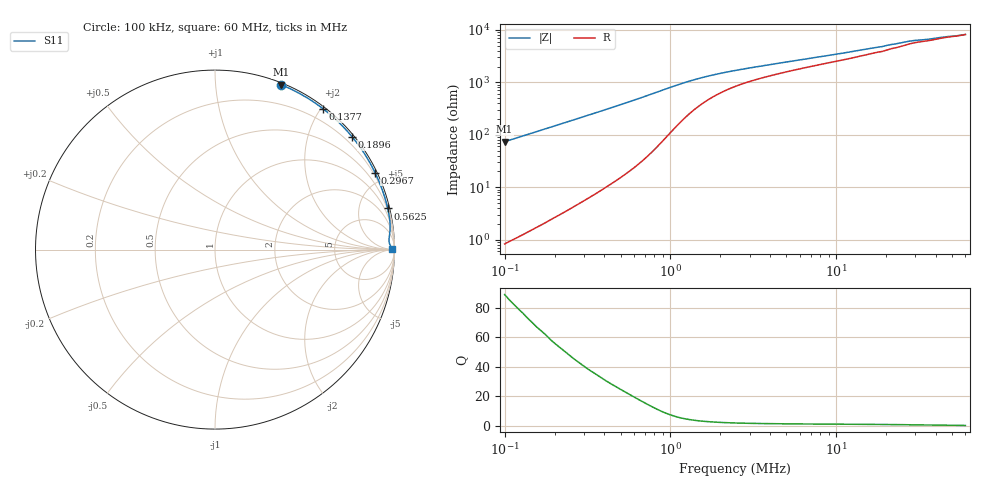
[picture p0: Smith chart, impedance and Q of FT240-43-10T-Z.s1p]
! ListType=Log
!!FT240-43 10T Z
# MHz S RI R 50
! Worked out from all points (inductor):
!   101 points, 100 kHz to 60 MHz, reference 50 ohm
!   read as one part to ground: L = 117 uH near 100 kHz
!   highest Q = 89 at 100 kHz (marker M1), where L = 117 uH
!   S11 on the Smith chart (normalised r, x): 100 kHz: 0.02, +1.47; 137.7 kHz: 0.03, +2.03; 189.6 kHz: 0.05, +2.79; 296.7 kHz: 0.11, +4.38; 562.5 kHz: 0.40, +8.48; 60 MHz: open
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0.1  0.3658 0.9195
0.1136483  0.4694 0.8709
0.1211559  0.5168 0.8436
0.1376916  0.6024 0.7846
0.1564842  0.6759 0.7222
0.1668215  0.7082 0.6906
0.1895899  0.7646 0.6276
0.2021141  0.7889 0.5968
0.2296993  0.8308 0.5372
0.2610494  0.8646 0.481
0.2966783  0.8917 0.4288
0.3371699  0.9133 0.3809
0.3831879  0.9303 0.3371
0.4354866  0.9437 0.2975
0.5276177  0.9585 0.2452
0.5624719  0.9622 0.2295
0.6814679  0.9705 0.187
0.8256385  0.9749 0.1508
1.00031  0.9757 0.1207
1.136835  0.9749 0.1042
1.377343  0.9729 0.0846
1.668732  0.9711 0.0699
2.021767  0.97 0.0587
2.611302  0.9697 0.0477
5.626461  0.9742 0.0281
12.92394  0.9808 0.0162
27.84666  0.9856 0.00738
60  0.9879 0.000776
